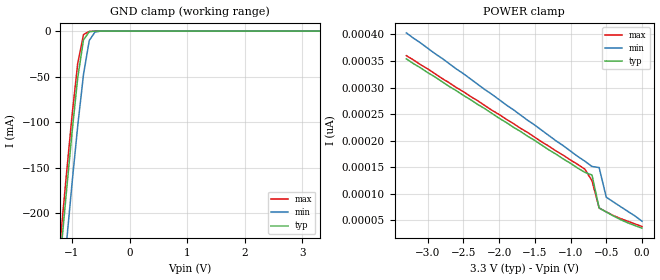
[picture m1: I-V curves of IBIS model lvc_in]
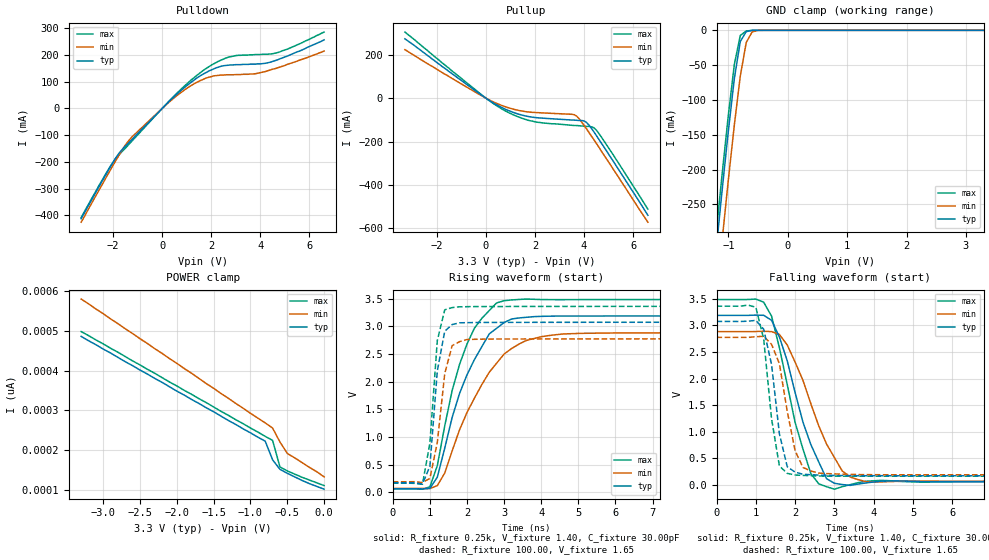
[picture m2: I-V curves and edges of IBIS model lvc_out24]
| IBIS file 16344x.ibs created by s2ibis2 version 1.1
| North Carolina State University Electronics Research Laboratory  1995
[IBIS ver]   2.1
[File name]   16344x.ibs
[File Rev]   1.0
[Date]   03/01/99 rtk
[Source]   Integrated Device Technology, Inc.
[Notes]   1.Temperatures: typ=25C, min=100C, max=0C 2.RRmp rates based
   on 50 ohm load.
[Disclaimer] Integrated Device Technology, Inc. ("IDT") hereby grants the
   user of this IBIS model a non-exclusive, nontransferable
   license to use this IBIS model under the following terms. The
   user is granted this license only to use the IBIS model and is
   not granted rights to sell, copy (except as needed to run the
   IBIS model), rent, lease or sub-license the IBIS model in
   whole or in part, or in modified form to anyone. The User may
   modify the IBIS model to suit its specific applications, but
   rights to derivative works and such modifications shall belong
   to IDT. This IBIS model is provided on an AS IS" basis and IDT
   makes absolutely no warranty with respect to the information
   contained herein. IDT DISCLAIMS AND CUSTOMER WAIVES ALL
   WARRANTIES, EXPRESS AND IMPLIED, INCLUDING WARRANTIES OF
   MERCHANTABILITY AND FITNESS FOR A PARTICULAR PURPOSE. THE
   ENTIRE RISK AS TO QUALITY AND PERFORMANCE IS WITH THE USER
   ACCORDINGLY, IN NO EVENT SHALL IDT BE LIABLE FOR ANY DIRECT OR
   INDIRECT DAMAGES, WHETHER IN CONTRACT OR TORT, INCLUDING ANY
   LOST PROFITS OR OTHER INCIDENTAL, CONSEQUENTIAL, EXEMPLARY, OR
   PUNITIVE DAMAGES ARISING OUT OF THE USE OR APPLICATION OF THE
   IBIS model. Further, IDT reserves the right to make changes
   without notice to any product herein to improve reliability,
   function, or design. IDT does not convey any license under
   patent rights or any other intellectual property rights,
   including those of third parties. IDT is not obligated to
   provide maintenance or support for the licensed IBIS model.
[Copyright]   Copyright 1997, Integrated Device Technology, Inc. all rights
   reserved
|   Component LVC16344A
[Component]   LVC16344A
[Manufacturer]   Integrated Device Technology
[Package]
| PA56
| variable   typ   min   max
R_pkg   6.50m   5.00m   10.00m
L_pkg   3.30nH   2.50nH   4.90nH
C_pkg   0.29pF   0.010pF   1.16pF
[Pin]  signal_name   model_name   R_pin   L_pin   C_pin
1   OE1B   lvc_in
2   B11   lvc_out24
3   B12   lvc_out24
4   GND   GND
5   B13   lvc_out24
6   B14   lvc_out24
7   VCC   POWER
8   A1   lvc_in
9   B21   lvc_out24
10   B22   lvc_out24
11   GND   GND
12   B23   lvc_out24
13   B24   lvc_out24
14   A2   lvc_in
15   A3   lvc_in
16   B31   lvc_out24
17   B32   lvc_out24
18   GND   GND
19   B33   lvc_out24
20   B34   lvc_out24
21   A4   lvc_in
22   VCC   POWER
23   B41   lvc_out24
24   B42   lvc_out24
25   GND   GND
26   B43   lvc_out24
27   B44   lvc_out24
28   OE2B   lvc_in
29   OE3B   lvc_in
30   B54   lvc_out24
31   B53   lvc_out24
32   GND   GND
33   B52   lvc_out24
34   B51   lvc_out24
35   VCC   POWER
36   A5   lvc_in
37   B64   lvc_out24
38   B63   lvc_out24
39   GND   GND
40   B62   lvc_out24
41   B61   lvc_out24
42   A6   lvc_in
43   A7   lvc_in
44   B74   lvc_out24
45   B73   lvc_out24
46   GND   GND
47   B72   lvc_out24
48   B71   lvc_out24
49   A8   lvc_in
50   VCC   POWER
51   B84   lvc_out24
52   B83   lvc_out24
53   GND   GND
54   B82   lvc_out24
55   B81   lvc_out24
56   OE4B   lvc_in
| Models and submodels in the file (2): lvc_in (Input), lvc_out24 (3-state)
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| in   in   dummy_model
| oe   oe   dummy_model
|   Model lvc_in
[Model]   lvc_in
Model_type   Input
Vinl =  0.800V
Vinh =  2.000V
C_comp   3.00pF   NA   NA
[Temperature Range]   25.00   100.00   0.000
[Voltage Range]   3.30V   3.00V   3.60V
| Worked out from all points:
|   GND clamp passes 1 mA (typ) near -0.70 V on its own axis
[GND_clamp]
| voltage   I(typ)   I(min)   I(max)
-3.3V     -1.806A    -1.858A    -1.789A
-1.2V     -248mA     -306mA     -229mA
-1.1V     -179mA     -236mA     -160mA
-1V       -112mA     -168mA     -93.56mA
-900mV    -51.39mA   -104mA     -35.36mA
-800mV    -9.697mA   -47.7mA    -3.786mA
-700mV    -714uA     -10.4mA    -348uA
-600mV    -52.42uA   -951uA     -8.225uA
-500mV    -126nA     -30.48uA   -10.89nA
3.3V      34.69pA    75.27pA    23pA
[POWER_clamp]
| voltage   I(typ)   I(min)   I(max)
-3.3V     354pA      403pA      360pA
-800mV    140pA      161pA      146pA
-700mV    135pA      151pA      124pA
-600mV    72.75pA    149pA      72.79pA
-500mV    65.09pA    93.05pA    65.39pA
-300mV    50.77pA    75.27pA    52.78pA
0V        34.68pA    47.91pA    37.83pA
|   Model lvc_out24
[Model]   lvc_out24
Model_type   3-state
Polarity   Non-Inverting
Enable   Active-High
Vinl =  0.000V
Vinh =  2.000V
Vmeas =  1.500V
C_comp   3.00pF   NA   NA
[Temperature Range]   25.00   100.00   0.000
[Voltage Range]   3.30V   3.00V   3.60V
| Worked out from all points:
|   slope of the pulldown table from 0 to 0.495 V, typ, clamps not added: 11.1 ohm
|   slope of the pullup table from 0 to 0.495 V, typ, clamps not added: 14.5 ohm
|   GND clamp passes 1 mA (typ) near -0.65 V on its own axis
|   rising waveform, R_fixture 0.25k, V_fixture 1.40, C_fixture 30.00pF: 20-80 % time 982ps typ, 1.24ns min, 811ps max; typ from 0.061 V to 3.19 V
|   rising waveform, R_fixture 100.00, V_fixture 1.65: 20-80 % time 251ps typ, 304ps min, 220ps max; typ from 0.171 V to 3.08 V
|   falling waveform, R_fixture 0.25k, V_fixture 1.40, C_fixture 30.00pF: 20-80 % time 747ps typ, 915ps min, 646ps max; typ from 3.19 V to 0.061 V
|   falling waveform, R_fixture 100.00, V_fixture 1.65: 20-80 % time 336ps typ, 378ps min, 296ps max; typ from 3.08 V to 0.171 V
[Pulldown]
| voltage   I(typ)   I(min)   I(max)
-3.3V     -413mA     -426mA     -409mA
-2.1V     -217mA     -229mA     -215mA
-1.8V     -173mA     -182mA     -178mA
-1.4V     -132mA     -125mA     -139mA
100mV     9.36mA     8.53mA     9.88mA
900mV     77.5mA     68.6mA     83.2mA
1.8V      135mA      114mA      150mA
2.6V      161mA      126mA      189mA
3.7V      166mA      129mA      201mA
4.4V      173mA      144mA      204mA
5.1V      196mA      165mA      222mA
6.6V      257mA      215mA      286mA
[Pullup]
| voltage   I(typ)   I(min)   I(max)
-3.3V     273mA      223mA      304mA
-200mV    15.7mA     12.6mA     17.8mA
800mV     -51.2mA    -39.9mA    -59.2mA
1.4V      -75.9mA    -58mA      -89.7mA
2V        -89.2mA    -66.1mA    -109mA
3.5V      -101mA     -74.3mA    -125mA
3.7V      -102mA     -83mA      -126mA
4.1V      -112mA     -141mA     -130mA
4.4V      -155mA     -191mA     -136mA
4.5V      -172mA     -208mA     -147mA
5.2V      -292mA     -329mA     -263mA
6.6V      -539mA     -571mA     -511mA
[GND_clamp]
| voltage   I(typ)   I(min)   I(max)
-3.3V     -2.206A    -2.271A    -2.184A
-1.2V     -310mA     -382mA     -286mA
-1.1V     -225mA     -297mA     -202mA
-1V       -144mA     -214mA     -121mA
-900mV    -69.29mA   -136mA     -48.96mA
-800mV    -16.14mA   -65.88mA   -7.431mA
-700mV    -1.8mA     -17.54mA   -933uA
-600mV    -143uA     -2.267mA   -21.88uA
-500mV    -316nA     -75.99uA   -26.99nA
3.3V      101pA      168pA      89pA
[POWER_clamp]
| voltage   I(typ)   I(min)   I(max)
-3.3V     486pA      580pA      498pA
-800mV    222pA      268pA      234pA
-700mV    175pA      255pA      224pA
-600mV    151pA      220pA      157pA
-500mV    141pA      191pA      147pA
-300mV    123pA      168pA      131pA
0V        101pA      132pA      110pA
[Ramp]
| variable   typ   min   max
dV/dt_r   1.45/0.32n   1.21/0.34n   1.64/0.23n
dV/dt_f   1.59/0.39n   1.41/0.50n   1.76/0.35n
R_load = 50.00
[Rising Waveform]
R_fixture = 0.25k
V_fixture = 1.40
C_fixture = 30.00pF
R_dut = 7.00m
L_dut = 3.30nH
C_dut = 0.29pF
| time   V(typ)   V(min)   V(max)
0s        61.33mV    67.59mV    57.9mV
1ns       68.18mV    64.46mV    95.45mV
1.2ns     271mV      118mV      480mV
1.4ns     796mV      346mV      1.199V
1.6ns     1.353V     747mV      1.841V
2ns       2.123V     1.442V     2.681V
2.6ns     2.864V     2.17V      3.286V
3ns       3.069V     2.5V       3.464V
4.6ns     3.186V     2.863V     3.483V
19.8ns    3.189V     2.884V     3.487V
[Rising Waveform]
R_fixture = 100.00
V_fixture = 1.65
R_dut = 7.00m
L_dut = 3.30nH
C_dut = 0.29pF
| time   V(typ)   V(min)   V(max)
0s        171mV      188mV      162mV
600ps     171mV      189mV      159mV
800ps     145mV      174mV      142mV
1ns       470mV      249mV      885mV
1.2ns     2.193V     898mV      2.744V
1.4ns     2.912V     2.145V     3.3V
1.6ns     3.033V     2.652V     3.34V
2ns       3.067V     2.762V     3.356V
2.6ns     3.071V     2.77V      3.359V
19.8ns    3.075V     2.775V     3.362V
[Falling Waveform]
R_fixture = 0.25k
V_fixture = 1.40
C_fixture = 30.00pF
R_dut = 7.00m
L_dut = 3.30nH
C_dut = 0.29pF
| time   V(typ)   V(min)   V(max)
0s        3.189V     2.884V     3.487V
1ns       3.194V     2.885V     3.496V
1.4ns     3.097V     2.883V     3.176V
1.8ns     2.332V     2.631V     1.885V
2.4ns     759mV      1.527V     214mV
2.8ns     115mV      768mV      -35.65mV
3ns       29.9mV     514mV      -81.29mV
3.4ns     -10.27mV   148mV      3.984mV
4ns       54.08mV    51.85mV    76.18mV
19.8ns    61.33mV    67.6mV     57.91mV
[Falling Waveform]
R_fixture = 100.00
V_fixture = 1.65
R_dut = 7.00m
L_dut = 3.30nH
C_dut = 0.29pF
| time   V(typ)   V(min)   V(max)
0s        3.075V     2.775V     3.362V
1ns       3.095V     2.788V     3.342V
1.2ns     2.928V     2.795V     2.746V
1.4ns     2.266V     2.644V     1.244V
1.6ns     960mV      2.279V     356mV
1.8ns     340mV      1.382V     216mV
2ns       239mV      641mV      185mV
2.2ns     199mV      327mV      178mV
2.6ns     183mV      221mV      166mV
19.8ns    171mV      188mV      162mV
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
